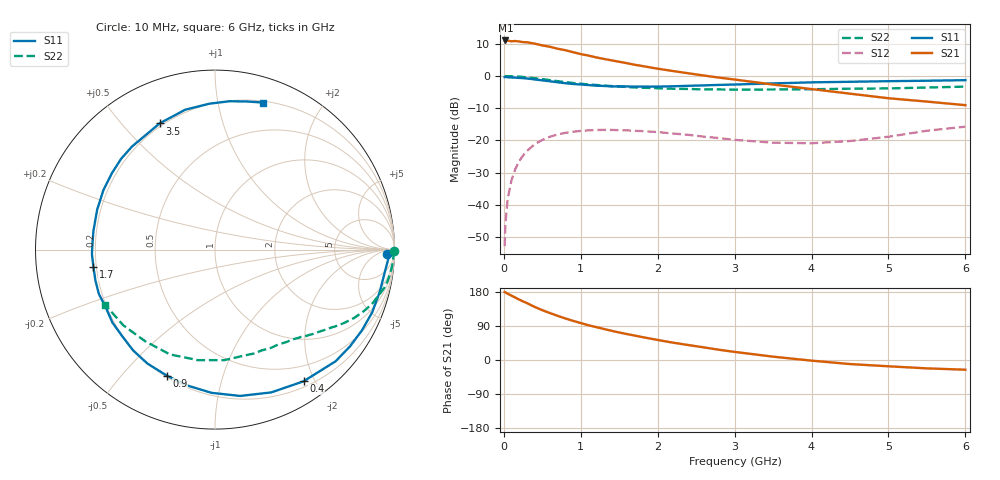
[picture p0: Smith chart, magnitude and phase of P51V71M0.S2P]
! SIEMENS Small Signal Semiconductors
! BFP183
! Si NPN RF Bipolar Junction Transistor in SOT143
! VCE = 1.75 V  IC = 1 mA
! Common Emitter S-Parameters:  March  1996
# GHz  S  MA  R  50
!  f  S11  S21  S12  S22
! GHz  MAG  ANG  MAG  ANG  MAG  ANG  MAG  ANG
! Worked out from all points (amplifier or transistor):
!   36 points, 10 MHz to 6 GHz, reference 50 ohm
!   highest |S21| = 11.0 dB at 20 MHz (marker M1)
!   |S21| within 3 dB of that: start of sweep to 795.1 MHz
!   unconditionally stable (mu >= 1): 2.462 GHz to end of sweep
!   at 250 MHz: K = 0.10, MSG = 17.6 dB, |S12| = -24.7 dB
!   at 1.4 GHz: K = 0.55, MSG = 10.8 dB, |S12| = -16.7 dB
!   at 6 GHz: K = 1.08, MAG = 1.6 dB, |S12| = -15.7 dB
!   S11 on the Smith chart (normalised r, x): 10 MHz: 38, -22; 400 MHz: 0.27, -1.85; 900 MHz: 0.21, -0.67; 1.7 GHz: 0.19, -0.07; 3.5 GHz: 0.19, +0.64; 6 GHz: 0.21, +1.35
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0.01  0.9611 -1.3  3.488 179.4  0.0023 89.3  0.9999 -0.5
0.02  0.9674 -2.9  3.556 178.6  0.005 85.7  0.9946 -1.0
0.05  0.9549 -7.3  3.527 174.9  0.0124 87.4  0.9947 -2.6
0.1  0.9477 -14.4  3.453 169.8  0.0244 80.5  0.991 -5.2
0.15  0.943 -21.8  3.485 164.6  0.0363 76.7  0.9846 -7.8
0.25  0.9255 -35.6  3.351 154.5  0.0585 68.3  0.9668 -12.7
0.3  0.9158 -42.8  3.332 150.2  0.0688 64.2  0.9516 -14.9
0.4  0.8843 -56.1  3.178 140.2  0.0873 56.7  0.9246 -19.3
0.5  0.8551 -68.5  2.98 131.5  0.1021 49.5  0.8928 -23.0
0.6  0.8272 -80.3  2.836 123.8  0.1144 43.2  0.8623 -26.3
0.7  0.7982 -91.4  2.646 116.5  0.124 37.3  0.8317 -29.2
0.8  0.7726 -101.6  2.511 109.6  0.1314 32.2  0.8048 -31.7
0.9  0.7516 -110.9  2.338 103.3  0.1367 27.5  0.7784 -34.0
1.1  0.7238 -129.1  2.072 91.7  0.1436 19.4  0.7401 -38.1
1.4  0.6883 -152.3  1.748 77.1  0.146 9.5  0.6983 -43.6
1.7  0.6842 -171.9  1.494 64.5  0.1412 2.6  0.6638 -48.7
2.2  0.6932 161.2  1.193 45.7  0.1283 -5.3  0.6338 -57.2
2.8  0.7278 135.9  0.943 26.9  0.109 -8.4  0.6187 -69.1
3.5  0.7679 113.7  0.737 8.8  0.0925 -1.3  0.618 -85.2
4.5  0.8134 92.3  0.532 -10.7  0.0981 17.2  0.6355 -113.3
5.5  0.8445 77.7  0.401 -22.1  0.1417 24.4  0.6625 -140.4
6  0.8615 72.0  0.353 -25.6  0.1639 21.6  0.6845 -153.2
